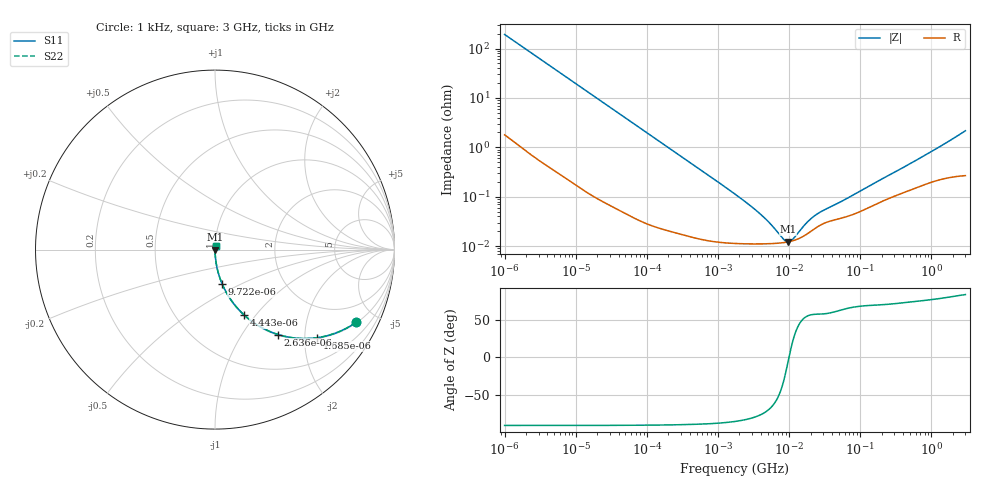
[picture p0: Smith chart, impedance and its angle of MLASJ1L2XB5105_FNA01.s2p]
! MLASJ1L2XB5105_FNA01  S-PARAMETER MODEL  ( Standard Model )
! Model Generated by TAIYO YUDEN Corporation (http://www.ty-top.com)
! Version 2.0
! TAIYO YUDEN Control No. 230320
! Copyright(c) 2011 TAIYO YUDEN CO.,LTD. All Rights Reserved.
! Product Description (link to TY-COMPAS)
! https://ds.yuden.co.jp/TYCOMPAS/or/detail?pn=MLASJ1L2XB5105MFNA01&u=M
! Products Name : Multilayer Ceramic Capacitors
! Characteristics :
!  Capacitance : 1 [uF] , Rated Voltage : 6.3 [V] , TCC : X5R
!  Case Size : 1.0 x 0.5 / 0.039 x 0.02 [mm/inch] , Thickness : 0.2 / 0.008 [mm/inch]
!  (Conditions: Temperature = 25 [degC] , DC Bias Voltage = 0 [V])
! External Node Assignments :
!  1  o---| |---o  2
! GND o---------o GND
! Frequency Range : 1kHz  -  3GHz  [ 401 STEP ]
# MHZ S RI R 50
! Freq[MHz].  S11 Real  S11 Imag  S21 Real  S21 Imag  S12 Real  S12 Imag  S22 Real  S22 Imag
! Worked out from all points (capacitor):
!   401 points, 1 kHz to 3 GHz, reference 50 ohm
!   read as one part in series: C = 825 nF near 1.077 kHz
!   lowest |Z| = 12.2 mohm at 9.626 MHz (marker M1)
!   series resonance near 9.938 MHz, so ESL is about 310 pH
!   S11 on the Smith chart (normalised r, x): 1 kHz: 1.04, -3.85; 1.685 kHz: 1.02, -2.29; 2.636 kHz: 1.01, -1.47; 4.443 kHz: 1.01, -0.87; 9.722 kHz: 1.00, -0.40; 3 GHz: 1.01, +0.04
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0.001  0.7854 -0.4059  0.2146 0.4059  0.2146 0.4059  0.7854 -0.4059
0.001685  0.5671 -0.4911  0.4329 0.4911  0.4329 0.4911  0.5671 -0.4911
0.002636  0.3515 -0.4732  0.6485 0.4732  0.6485 0.4732  0.3515 -0.4732
0.004443  0.1624 -0.3645  0.8376 0.3645  0.8376 0.3645  0.1624 -0.3645
0.006451  0.0853 -0.275  0.9147 0.275  0.9147 0.275  0.0853 -0.275
0.009722  0.0402 -0.1921  0.9598 0.1921  0.9598 0.1921  0.0402 -0.1921
0.01216  0.0264 -0.156  0.9736 0.156  0.9736 0.156  0.0264 -0.156
0.033275  0.00407 -0.0587  0.9959 0.0587  0.9959 0.0587  0.00407 -0.0587
0.147855  0.00041 -0.0134  0.9996 0.0134  0.9996 0.0134  0.00041 -0.0134
1.732051  0.000114 -0.00112  0.9999 0.00112  0.9999 0.00112  0.000114 -0.00112
3.93371  0.000111 -0.000432  0.9999 0.000432  0.9999 0.000432  0.000111 -0.000432
5.502215  0.000112 -0.000255  0.9999 0.000255  0.9999 0.000255  0.000112 -0.000255
8.291982  0.000118 -7.44e-05  0.9999 7.44e-05  0.9999 7.44e-05  0.000118 -7.44e-05
9.625639  0.000122 -1.31e-05  0.9999 1.31e-05  0.9999 1.31e-05  0.000122 -1.31e-05
11.1738  0.000128 4.82e-05  0.9999 -4.82e-05  0.9999 -4.82e-05  0.000128 4.82e-05
16.83921  0.000167 0.000221  0.9998 -0.000221  0.9998 -0.000221  0.000167 0.000221
21.06097  0.000208 0.000314  0.9998 -0.000314  0.9998 -0.000314  0.000208 0.000314
28.38055  0.000273 0.000424  0.9997 -0.000424  0.9997 -0.000424  0.000273 0.000424
57.63471  0.000378 0.000751  0.9996 -0.000751  0.9996 -0.000751  0.000378 0.000751
256.0921  0.000937 0.00258  0.9991 -0.00258  0.9991 -0.00258  0.000937 0.00258
980.2507  0.002 0.00783  0.998 -0.00783  0.998 -0.00783  0.002 0.00783
3000  0.00313 0.0214  0.9969 -0.0214  0.9969 -0.0214  0.00313 0.0214
